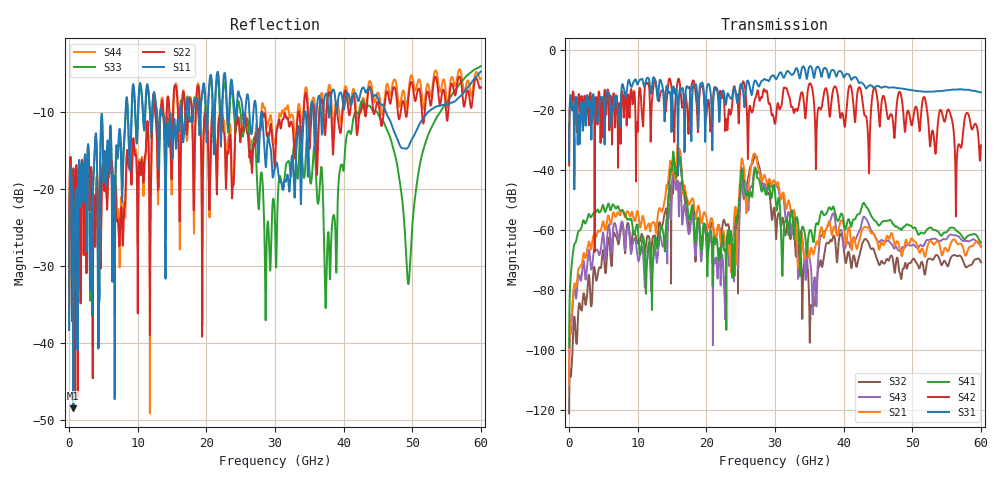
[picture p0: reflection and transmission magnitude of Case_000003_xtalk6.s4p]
! Info: Touchstone file created by circ.  Input file=CasetestDOE_NRZ_template_000003.circ
# Hz S RI R 50
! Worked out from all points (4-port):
!   6000 points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, 10 MHz to 60 GHz, reference 50 ohm
!   strongest paths, dB at 10 MHz, 15.01 GHz, 30.01 GHz, 45.01 GHz, 60 GHz:
!     S31: -37.2, -18.2, -9.3, -12.0, -14.1
!     S42: -38.6, -14.8, -24.6, -18.3, -31.8
!     S41: -98.9, -39.3, -47.6, -58.3, -64.3
!     S21: -111.6, -39.6, -44.2, -65.0, -65.8
!     S43: -111.5, -43.6, -44.8, -64.0, -65.4
!     S32: -121.2, -46.7, -55.1, -70.8, -70.8
!   lowest |S11| = -48.5 dB at 610 MHz (marker M1), VSWR 1.01, Z = 50.4 - j0.00327 ohm
!   |S11| at or under -10 dB: start of sweep to 8.238 GHz; 27.29 GHz to 34.34 GHz (7.049 GHz wide, 22.9 % of centre); 46.15 GHz to 52.31 GHz (6.159 GHz wide, 12.5 % of centre)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
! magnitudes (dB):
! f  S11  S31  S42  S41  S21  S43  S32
! 10 MHz  -38.3  -37.2  -38.6  -98.9  -111.6  -111.5  -121.2
! 610 MHz  -48.5  -18.7  -13.8  -67.0  -81.7  -81.6  -93.2
! 12.08 GHz  -11.6  -12.1  -16.9  -85.7  -57.7  -74.3  -64.5
! 15.98 GHz  -12.3  -17.6  -9.6  -37.0  -33.1  -54.5  -33.8
! 27.23 GHz  -9.3  -10.4  -15.6  -40.3  -35.4  -40.0  -35.2
! 35.23 GHz  -9.2  -5.5  -11.4  -60.2  -66.1  -72.6  -85.8
! 60 GHz  -4.7  -14.1  -31.8  -64.3  -65.8  -65.4  -70.8
